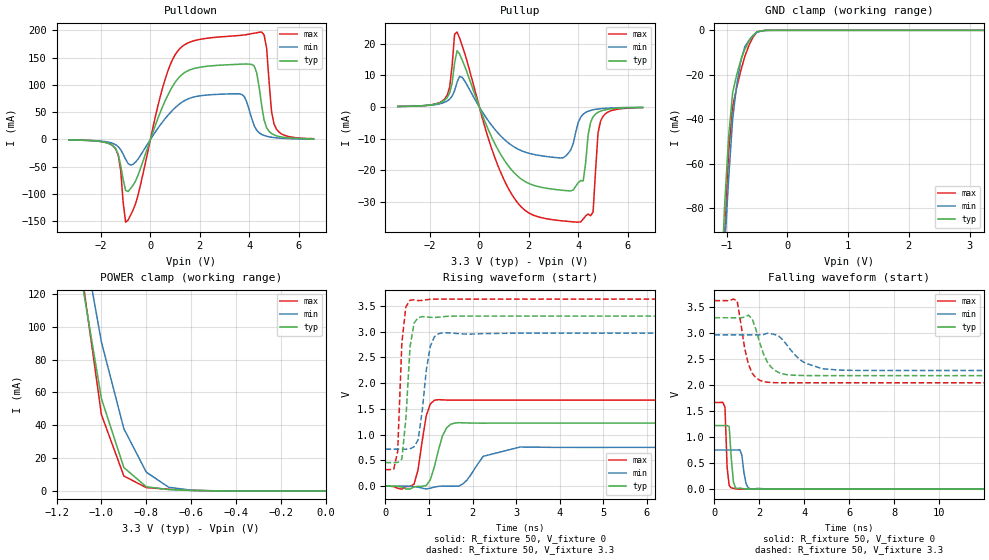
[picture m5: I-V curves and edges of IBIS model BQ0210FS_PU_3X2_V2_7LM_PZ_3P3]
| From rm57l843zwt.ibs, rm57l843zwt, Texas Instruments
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|   Model Cell BQ0210FS_PU_3X2_V2_7LM_PZ_3P3
|BQ0210FS_PU_3X2_V2_7LM_PZ_3P3
[Model]   BQ0210FS_PU_3X2_V2_7LM_PZ_3P3
Model_type   I/O
Polarity   Non-Inverting
Enable   Active-Low
Vinl =  1.15
Vinh =  1.55
Cref =  15.0001pF
Rref =  101.0000M
Vref =  0V
Vmeas =  1.65
C_comp   1.2p   1.2p   1.2p
[Model Spec]
Vinl   1.15   1.02   1.28
Vinh   1.55   1.45   1.65
[Temperature Range]   25   155   -40
[Voltage Range]   3.3   2.97   3.63
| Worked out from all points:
|   slope of the pulldown table from 0 to 0.495 V, typ, clamps not added: 8.21 ohm
|   slope of the pullup table from 0 to 0.495 V, typ, clamps not added: 52.1 ohm
|   GND clamp passes 1 mA (typ) near -0.51 V on its own axis
|   POWER clamp passes 1 mA (typ) near -0.71 V on its own axis
|   rising waveform, R_fixture 50, V_fixture 0: 20-80 % time 237ps typ, 451ps min, 180ps max; typ from 0 V to 1.22 V
|   rising waveform, R_fixture 50, V_fixture 3.3: 20-80 % time 134ps typ, 196ps min, 106ps max; typ from 0.458 V to 3.3 V
|   falling waveform, R_fixture 50, V_fixture 0: 20-80 % time 132ps typ, 152ps min, 96.8ps max; typ from 1.22 V to 0 V
|   falling waveform, R_fixture 50, V_fixture 3.3: 20-80 % time 29.5ns typ, 31.8ns min, 18.4ns max; typ from 3.3 V to 0.465 V
[POWER_clamp]
|   voltage   I(typ)   I(min)   I(max)
-3.3V     2.37A      2.626A     3.145A
-1.1V     138.4mA    167.6mA    144.7mA
-1.067V   111mA      142mA      112mA
-1.033V   83.64mA    116.3mA    79.23mA
-1V       56.26mA    90.72mA    46.48mA
-900mV    14.22mA    37.92mA    9.099mA
-800mV    2.537mA    11.42mA    2.002mA
-700mV    806.6uA    2.223mA    1.026mA
-600mV    280.6uA    454.5uA    364.3uA
-500mV    47.71uA    99.18uA    51.8uA
0V        413.5pA    9.276nA    341.9pA
[Pulldown]
|   voltage   I(typ)   I(min)   I(max)
-3.3V     -899.6uA   -820.6uA   -837.7uA
-1.4V     -17.27mA   -9.734mA   -17.51mA
-1.2V     -47.62mA   -18.77mA   -56.87mA
-1V       -93.34mA   -36.32mA   -151.7mA
1.1V      110.9mA    62.27mA    162mA
3.6V      138mA      83.62mA    190.9mA
4.1V      137.6mA    38.13mA    194.2mA
4.5V      62.69mA    9.297mA    197.1mA
4.7V      21.72mA    5.946mA    167.7mA
4.9V      10.98mA    4.145mA    51.34mA
5.1V      6.781mA    3.055mA    18.84mA
6.6V      1.042mA    806uA      1.545mA
[Pullup]
|   voltage   I(typ)   I(min)   I(max)
-3.3V     154uA      152.3uA    178.5uA
-1.4V     2.171mA    1.484mA    2.544mA
-900mV    17.81mA    7.857mA    23.72mA
500mV     -9.587mA   -5.844mA   -13.22mA
1.4V      -20.78mA   -12.62mA   -28.76mA
3.4V      -26.42mA   -16.07mA   -36.11mA
4V        -23.95mA   -4.859mA   -36.5mA
4.2V      -23.43mA   -2.288mA   -35.5mA
4.6V      -3.136mA   -899.4uA   -33.27mA
4.8V      -1.694mA   -637.7uA   -8.23mA
5V        -1.071mA   -474.1uA   -2.98mA
6.6V      -155uA     -124.4uA   -196.9uA
[GND_clamp]
|   voltage   I(typ)   I(min)   I(max)
-3.3V     -1.949A    -1.625A    -3.258A
-1.1V     -122.2mA   -133.9mA   -153mA
-1.033V   -79.16mA   -98.31mA   -94.35mA
-966.7mV  -47.74mA   -66.91mA   -54.79mA
-900mV    -27.95mA   -39.72mA   -34.29mA
-833.3mV  -19.95mA   -24.6mA    -25.69mA
-766.7mV  -13.45mA   -13.82mA   -18.17mA
-700mV    -8.461mA   -7.363mA   -11.74mA
-566.7mV  -2.389mA   -2.348mA   -3.171mA
-500mV    -626.6uA   -897.7uA   -720.6uA
-300mV    -1.304uA   -11.25uA   -644.9nA
3.233V    397.1pA    1.073uA    272.4pA
[Ramp]
| variable   typ   min   max
dV/dt_f   1.749664/29.50636n   0.5676662/0.3496601n   2.040351/18.38879n
dV/dt_r  0.7840602/0.2503309n  0.4913194/0.4100077n   1.053953/0.1904155n
R_load = 50
[Rising Waveform]
R_fixture = 50
V_fixture = 0
V_fixture_min = 0
V_fixture_max = 0
|   time   V(typ)   V(min)   V(max)
0s        -5.652uV   -4.008uV   -12.39uV
656ps     -14.38mV   -7.695mV   38.68mV
748ps     -1.348mV   -18.28mV   320.2mV
936ps     14.05mV    -54.18mV   1.368V
1.216ns   700.1mV    -3.508mV   1.678V
1.496ns   1.2V       -600.1uV   1.67V
1.872ns   1.227V     117.7mV    1.669V
2.244ns   1.223V     579.9mV    1.669V
3.092ns   1.224V     759.8mV    1.669V
35.53ns   1.224V     753.2mV    1.669V
[Rising Waveform]
R_fixture = 50
V_fixture = 3.3
V_fixture_min = 2.97
V_fixture_max = 3.63
|   time   V(typ)   V(min)   V(max)
0s        457.6mV    717.3mV    321.7mV
188ps     457.3mV    717.4mV    326.6mV
280ps     460.5mV    717.3mV    673.9mV
376ps     523mV      716.7mV    2.784V
468ps     1.304V     717mV      3.479V
564ps     2.707V     727.7mV    3.609V
748ps     3.269V     896.9mV    3.601V
1.028ns   3.276V     2.714V     3.627V
1.308ns   3.288V     2.975V     3.63V
35.53ns   3.3V       2.97V      3.63V
[Falling Waveform]
R_fixture = 50
V_fixture = 0
V_fixture_min = 0
V_fixture_max = 0
|   time   V(typ)   V(min)   V(max)
0s        1.224V     753.2mV    1.669V
468ps     1.225V     753.2mV    1.579V
564ps     1.225V     753.2mV    411.6mV
656ps     1.204V     753.2mV    67.98mV
844ps     138.6mV    753.4mV    17.02mV
1.028ns   11.77mV    753.8mV    2.675mV
1.216ns   13.59mV    659.5mV    671.1uV
1.404ns   3.294mV    104.7mV    939uV
1.684ns   507.3uV    -533.9uV   771.1uV
35.53ns   157.9uV    1.958uV    1.88uV
[Falling Waveform]
R_fixture = 50
V_fixture = 3.3
V_fixture_min = 2.97
V_fixture_max = 3.63
|   time   V(typ)   V(min)   V(max)
0s        3.3V       2.97V      3.63V
1.008ns   3.299V     2.97V      3.628V
1.512ns   3.35V      2.97V      2.4V
2.18ns    2.604V     2.977V     2.071V
18.06ns   2.185V     2.285V     2.051V
20.81ns   2.185V     2.285V     476.9mV
29.14ns   2.188V     2.285V     345mV
34.83ns   551.4mV    2.285V     344.8mV
35.93ns   525.4mV    755.6mV    344.8mV
36.81ns   465.4mV    755.6mV    344.8mV
